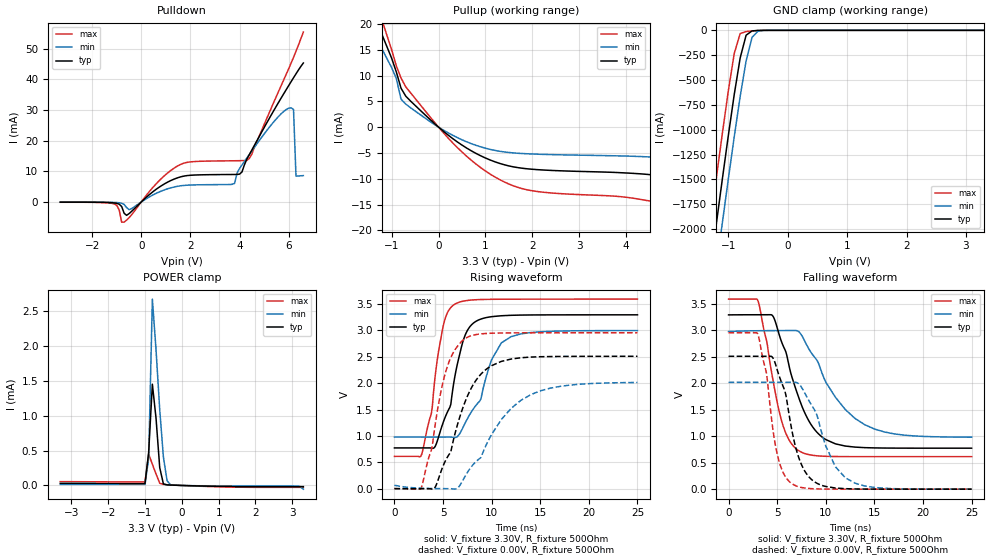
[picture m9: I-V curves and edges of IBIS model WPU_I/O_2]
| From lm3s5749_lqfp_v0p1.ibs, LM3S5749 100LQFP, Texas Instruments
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[Model]   WPU_I/O_2
Model_type   I/O
Vinl = 1.26
Vinh = 2.04
Vmeas = 1.65
| variable   typ   min   max
C_comp   9.739pF   9.739pF   9.803pF
[Model Spec]
Vinh+   1.91   1.78   2.04
Vinh-   1.90   1.76   2.03
Vinl+   1.40   1.27   1.54
Vinl-   1.39   1.26   1.53
| variable   typ   min   max
[Temperature Range]  25   85   -40
[Voltage Range]   3.3V   3.0V   3.6V
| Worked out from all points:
|   slope of the pulldown table from 0 to 0.495 V, typ, clamps not added: 143 ohm
|   slope of the pullup table from 0 to 0.495 V, typ, clamps not added: 143 ohm
|   GND clamp passes 1 mA (typ) near -0.48 V on its own axis
|   POWER clamp passes 1 mA (typ) near -0.71 V on its own axis
|   falling waveform, V_fixture 3.30V, R_fixture 500Ohm: 20-80 % time 2.85ns typ, 4.24ns min, 1.93ns max; typ from 3.29 V to 0.774 V
|   rising waveform, V_fixture 3.30V, R_fixture 500Ohm: 20-80 % time 1.99ns typ, 2.79ns min, 1.46ns max; typ from 0.774 V to 3.3 V
|   falling waveform, V_fixture 0.00V, R_fixture 500Ohm: 20-80 % time 1.94ns typ, 2.63ns min, 1.43ns max; typ from 2.51 V to 0 V
|   rising waveform, V_fixture 0.00V, R_fixture 500Ohm: 20-80 % time 3.04ns typ, 4.58ns min, 2ns max; typ from 0.005 V to 2.51 V
[Pulldown]
|  Voltage   I(typ)   I(min)   I(max)
-3.3V     -63.97uA   -36.29uA   -90.89uA
-1.1V     -317.2uA   -146.3uA   -639.5uA
-700mV    -3.674mA   -802.3uA   -6.562mA
-500mV    -3.8mA     -2.497mA   -5.142mA
1.6V      8.18mA     5.265mA    12.23mA
3.8V      8.962mA    6.06mA     13.43mA
4.1V      9.779mA    12.05mA    13.48mA
4.3V      13.99mA    14.33mA    13.54mA
6.1V      39.18mA    30.7mA     45.23mA
6.2V      40.48mA    30.1mA     47.14mA
6.3V      41.75mA    8.417mA    49.11mA
6.6V      45.28mA    8.602mA    55.36mA
[Pullup]
|  Voltage   I(typ)   I(min)   I(max)
-3.3V     58.84mA    18.65mA    75.09mA
-1.5V     24.39mA    20.24mA    28.75mA
-1.3V     20.01mA    16.77mA    23.31mA
-1.2V     17.8mA     15.03mA    20.55mA
-900mV    10.68mA    9.415mA    11.86mA
-800mV    7.542mA    5.414mA    9.524mA
-700mV    6.013mA    4.481mA    7.814mA
500mV     -3.481mA   -2.455mA   -4.825mA
1.5V      -7.517mA   -4.915mA   -11.03mA
5V        -9.793mA   -6.102mA   -15.25mA
6V        -12.34mA   -7.491mA   -19.35mA
6.6V      -15.07mA   -8.994mA   -23.96mA
[GND Clamp]
|  Voltage   I(typ)   I(min)   I(max)
-3.3V     -11.73A    -12.14A    -11.32A
-1.4V     -2.85A     -3.29A     -2.391A
-1.3V     -2.393A    -2.835A    -1.933A
-1.2V     -1.942A    -2.383A    -1.481A
-1.1V     -1.496A    -1.937A    -1.038A
-1V       -1.061A    -1.498A    -612.1mA
-900mV    -646.5mA   -1.071A    -233.9mA
-800mV    -278.2mA   -665.9mA   -32.19mA
-700mV    -49.13mA   -307.7mA   -12.51mA
-600mV    -5.771mA   -70.87mA   -6.526mA
-500mV    -1.221mA   -8.174mA   -2.28mA
3.3V      2.312nA    7.026uA    -6.841uA
[POWER Clamp]
|  Voltage   I(typ)   I(min)   I(max)
-3.3V     29.71uA    15.87uA    54.94uA
-1V       27.67uA    14.78uA    51.22uA
-900mV    477.6uA    387.3uA    449.4uA
-800mV    1.453mA    2.675mA    305uA
-700mV    962.1uA    1.944mA    163.7uA
-600mV    254.6uA    1.086mA    31.4uA
-500mV    22.38uA    405.6uA    14.49uA
-400mV    7.783uA    67.02uA    10.49uA
-300mV    5.498uA    7.026uA    7.722uA
3.1V      -16.64uA   -9.952uA   -27.43uA
3.2V      -16.65uA   -12.25uA   -27.44uA
3.3V      -16.65uA   -53.27uA   -27.45uA
[Ramp]
| variable   typ   min   max
dV/dt_f   1.51/2.85n   1.20/4.24n   1.79/1.93n
dV/dt_r   1.50/3.04n   1.17/4.58n   1.77/2.00n
R_load = 500Ohm
[Falling Waveform]
V_fixture = 3.30V
V_fixture_min = 3.00V
V_fixture_max = 3.60V
R_fixture = 500Ohm
|   Time   V(typ)   V(min)   V(max)
0s        3.293V     2.978V     3.591V
3ns       3.295V     2.993V     3.57V
4.5ns     3.284V     2.995V     2.131V
5.4ns     2.81V      2.996V     1.328V
7.2ns     1.741V     2.978V     729.6mV
8.4ns     1.246V     2.607V     647.5mV
9.7ns     974.5mV    2.152V     623.1mV
12ns      815mV      1.507V     615.1mV
14ns      784.7mV    1.219V     614.3mV
25ns      774.3mV    981.9mV    614.1mV
[Rising Waveform]
V_fixture = 3.30V
V_fixture_min = 3.00V
V_fixture_max = 3.60V
R_fixture = 500Ohm
|   Time   V(typ)   V(min)   V(max)
0s        774.3mV    980.2mV    614.1mV
2.8ns     774.3mV    980mV      649.9mV
3.8ns     770.2mV    980mV      1.426V
5ns       1.249V     979.9mV    3.068V
5.8ns     1.6V       979.6mV    3.434V
6.2ns     2.111V     973mV      3.496V
7.9ns     3.101V     1.453V     3.576V
10ns      3.261V     2.448V     3.59V
12ns      3.287V     2.883V     3.592V
25ns      3.296V     2.998V     3.594V
[Falling Waveform]
V_fixture = 0.00V
V_fixture_min = 0.00V
V_fixture_max = 0.00V
R_fixture = 500Ohm
|   Time   V(typ)   V(min)   V(max)
0s        2.51V      2.018V     2.956V
3ns       2.51V      2.018V     2.933V
3.9ns     2.51V      2.018V     2.19V
5ns       2.258V     2.018V     667.7mV
5.9ns     1.774V     2.018V     221mV
6.6ns     1.032V     2.019V     94.37mV
8.4ns     206.6mV    1.631V     11.33mV
11ns      21.52mV    421.7mV    712.2uV
12ns      9.312mV    217.6mV    301.3uV
25ns      30.04uV    131.8uV    20.33uV
[Rising Waveform]
V_fixture = 0.00V
V_fixture_min = 0.00V
V_fixture_max = 0.00V
R_fixture = 500Ohm
|   Time   V(typ)   V(min)   V(max)
0s        4.943mV    67.66mV    206.4uV
2.8ns     491.7uV    11.59mV    38.62mV
4.1ns     7.127mV    5.275mV    1.099V
5.3ns     550.3mV    2.605mV    2.232V
6.4ns     1.16V      2.695mV    2.679V
7.3ns     1.663V     245.8mV    2.849V
9.7ns     2.299V     928mV      2.945V
12ns      2.458V     1.522V     2.954V
14ns      2.495V     1.781V     2.955V
25ns      2.51V      2.014V     2.956V
